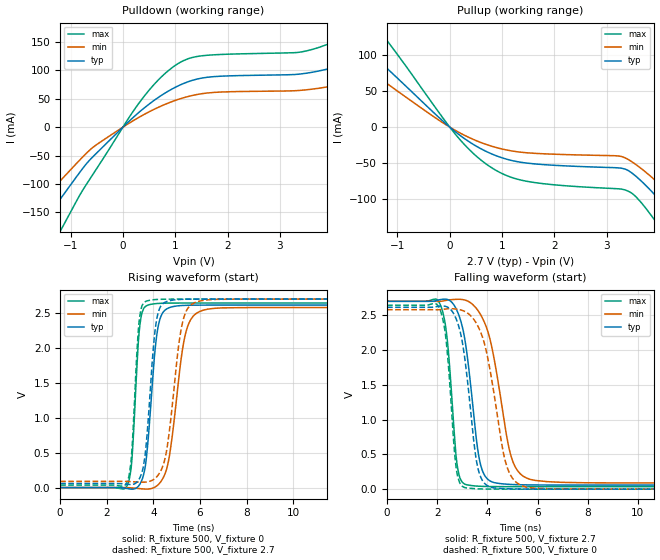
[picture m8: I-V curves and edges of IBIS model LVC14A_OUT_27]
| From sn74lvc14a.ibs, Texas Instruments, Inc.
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[Model]   LVC14A_OUT_27
Model_type  Output
Vref =   0
Rref =   500
Cref =   50p
Vmeas =   1.5
| variable   typ   min   max
C_comp   8.01pF   4.32pF   13.64pF
| C_pullup   6.96pF   4.39pF   8.24pF
| C_pulldown   9.05pF   4.32pF   13.64pF
[Temperature Range]   40   100   -40
| Ambient temperature   25   85   -40
[Voltage range]   2.7   2.7   2.7
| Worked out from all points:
|   slope of the pulldown table from 0 to 0.405 V, typ, clamps not added: 12 ohm
|   slope of the pullup table from 0 to 0.405 V, typ, clamps not added: 18.4 ohm
|   rising waveform, R_fixture 500, V_fixture 0: 20-80 % time 382ps typ, 575ps min, 257ps max; typ from 0 V to 2.61 V
|   falling waveform, R_fixture 500, V_fixture 2.7: 20-80 % time 517ps typ, 763ps min, 336ps max; typ from 2.7 V to 0.059 V
|   rising waveform, R_fixture 500, V_fixture 2.7: 20-80 % time 364ps typ, 541ps min, 252ps max; typ from 0.059 V to 2.7 V
|   falling waveform, R_fixture 500, V_fixture 0: 20-80 % time 505ps typ, 739ps min, 330ps max; typ from 2.61 V to 0 V
[Pulldown]
| LVC14A_OUT_27
|   Voltage   I(typ)   I(min)   I(max)
-5.5V     -612.9mA   -500.5mA   -770.2mA
-2.12V    -241.4mA   -186mA     -328.1mA
-1.585V   -175.5mA   -133.1mA   -246.9mA
-1.155V   -121.3mA   -90.3mA    -175.9mA
-565mV    -51.37mA   -35mA      -81.94mA
365mV     30.55mA    20.29mA    49.46mA
1.32V     82.21mA    55.61mA    122.5mA
3.86V     101.2mA    70.1mA     144mA
4.6V      122.9mA    85.26mA    177.9mA
5.865V    179.4mA    126.8mA    260.1mA
7.2V      255.1mA    185.8mA    363.1mA
11V       504.4mA    390.8mA    686.5mA
[Pullup]
| LVC14A_OUT_27
|   Voltage   I(typ)   I(min)   I(max)
-5.5V     374mA      297.8mA    508.8mA
-2.75V    187.4mA    144mA      265.3mA
-2.125V   145mA      110mA      208mA
-1.375V   93.79mA    69.84mA    137.3mA
60mV      -3.673mA   -2.608mA   -5.615mA
725mV     -34.79mA   -24.76mA   -52.84mA
1.475V    -50.05mA   -35.71mA   -75.37mA
3.375V    -59.06mA   -43.58mA   -88.01mA
4.03V     -102.9mA   -80.58mA   -140.9mA
4.465V    -140.4mA   -111.1mA   -189.1mA
4.865V    -177.6mA   -141.5mA   -236.5mA
11V       -824.7mA   -682.9mA   -1.028A
[Ramp]
| LVC14A_OUT_27
| variable   typ   min   max
dV/dt_r   1.58/3.95E-10   1.56/5.88E-10   1.60/2.71E-10
dV/dt_f   1.60/5.33E-10   1.58/7.77E-10   1.62/3.46E-10
R_load = 500
[Rising Waveform]
| LVC14A_OUT_27
R_fixture =   500
C_fixture =   0
L_fixture =   0
V_fixture =   0
V_fixture_min = 0
V_fixture_max = 0
|   Time   V(typ)   V(min)   V(max)
0s        178.1pV    3.672nV    17.91pV
2.87ns    -13.3mV    -462.3uV   27.09mV
3.07ns    -22.49mV   -4.328mV   374.8mV
3.435ns   58.13mV    -15.62mV   2.364V
3.685ns   389.2mV    -21.67mV   2.6V
3.975ns   1.581V     -7.327mV   2.63V
4.415ns   2.512V     137.9mV    2.64V
5.4ns     2.61V      2.233V     2.643V
6.335ns   2.614V     2.556V     2.643V
50ns      2.614V     2.579V     2.644V
[Falling Waveform]
| LVC14A_OUT_27
R_fixture =   500
C_fixture =   0
L_fixture =   0
V_fixture =   2.7
V_fixture_min = 2.7
V_fixture_max = 2.7
|   Time   V(typ)   V(min)   V(max)
0s        2.7V       2.7V       2.7V
2.115ns   2.724V     2.7V       2.659V
2.405ns   2.727V     2.716V     2.133V
2.815ns   2.544V     2.729V     301mV
3.325ns   1.521V     2.68V      54.15mV
3.64ns    510.6mV    2.559V     43.04mV
3.905ns   189.3mV    2.378V     39.17mV
4.97ns    67.36mV    443.5mV    36.1mV
5.9ns     60.54mV    126.1mV    35.96mV
50ns      58.93mV    88.64mV    35.94mV
[Rising Waveform]
| LVC14A_OUT_27
R_fixture =   500
C_fixture =   0
L_fixture =   0
V_fixture =   2.7
V_fixture_min = 2.7
V_fixture_max = 2.7
|   Time   V(typ)   V(min)   V(max)
0s        58.93mV    88.64mV    35.94mV
2.85ns    48.48mV    88.18mV    64.64mV
3.055ns   43.78mV    84.87mV    436.1mV
3.41ns    135.3mV    78.3mV     2.441V
3.65ns    486.1mV    78.66mV    2.661V
3.9ns     1.56V      97.27mV    2.686V
4.315ns   2.598V     239.9mV    2.696V
5.265ns   2.696V     2.386V     2.7V
6.095ns   2.7V       2.679V     2.7V
50ns      2.7V       2.7V       2.7V
[Falling Waveform]
| LVC14A_OUT_27
R_fixture =   500
C_fixture =   0
L_fixture =   0
V_fixture =   0
V_fixture_min = 0
V_fixture_max = 0
|   Time   V(typ)   V(min)   V(max)
0s        2.614V     2.579V     2.644V
2.095ns   2.631V     2.579V     2.594V
2.365ns   2.623V     2.59V      2.103V
2.77ns    2.433V     2.587V     269.1mV
3.185ns   1.624V     2.536V     17.49mV
3.54ns    460.6mV    2.396V     6.509mV
3.785ns   134.6mV    2.205V     3.103mV
4.765ns   6.352mV    339.6mV    174.5uV
5.66ns    1.175mV    21.49mV    15.27uV
50ns      1.072nV    15.52nV    513.6pV
